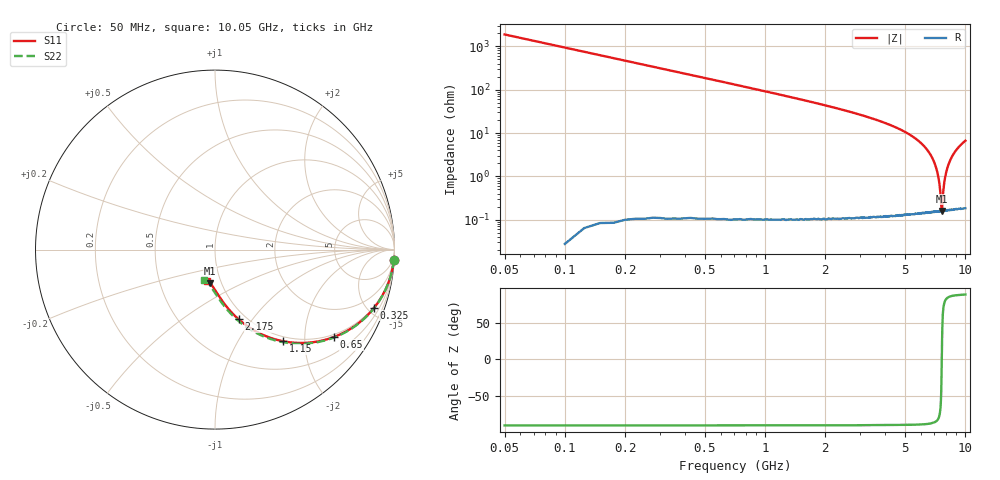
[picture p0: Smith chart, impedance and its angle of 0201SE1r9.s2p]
! AVX Thin Film Operation		Date: August 2001
! Description: Accu-P® Series, Thin Film, SMD, RF Capacitor
! Part Number: 02013J1R9ABW
! 50 MHz  -  10.05 GHz
! Serial Measurements
# mhz S db R 50
!	S11		S21		S12		S22
!	dB	Phase	dB	Phase	dB	Phase	dB	Phase
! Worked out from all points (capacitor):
!   401 points, 50 MHz to 10.05 GHz, reference 50 ohm
!   read as one part in series: C = 1.7 pF near 100 MHz
!   lowest |Z| = 159 mohm at 7.65 GHz (marker M1)
!   series resonance near 7.657 GHz, so ESL is about 250 pH
!   S11 on the Smith chart (normalised r, x): 50 MHz: 1, -36; 325 MHz: 0.92, -5.52; 650 MHz: 0.92, -2.77; 1.15 GHz: 0.92, -1.58; 2.175 GHz: 0.92, -0.86; 10.05 GHz: 0.86, -0.31
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50  -0.01 -3.2  -25.45 86.8  -25.45 86.8  -0.01 -3.2
75  -0.03 -4.8  -21.94 85.2  -21.94 85.2  -0.03 -4.8
125  -0.08 -7.9  -17.55 82.0  -17.55 82.0  -0.08 -8.0
175  -0.15 -11.1  -14.71 78.9  -14.71 78.9  -0.15 -11.1
250  -0.30 -15.6  -11.76 74.3  -11.76 74.3  -0.30 -15.7
325  -0.50 -20.0  -9.68 69.9  -9.68 69.9  -0.50 -20.2
400  -0.73 -24.2  -8.12 65.7  -8.12 65.7  -0.73 -24.4
475  -1.00 -28.1  -6.89 61.7  -6.89 61.7  -1.00 -28.4
650  -1.71 -36.4  -4.89 53.4  -4.89 53.4  -1.70 -36.7
875  -2.71 -45.1  -3.35 44.6  -3.35 44.6  -2.71 -45.6
1150  -3.94 -53.4  -2.25 36.2  -2.25 36.2  -3.94 -54.1
1425  -5.10 -59.8  -1.61 29.7  -1.61 29.7  -5.10 -60.6
1725  -6.25 -65.2  -1.19 24.2  -1.19 24.2  -6.25 -66.2
2175  -7.74 -71.3  -0.81 18.0  -0.81 18.0  -7.74 -72.5
2725  -9.23 -76.6  -0.56 12.4  -0.56 12.4  -9.23 -78.2
3400  -10.66 -81.5  -0.40 7.3  -0.40 7.3  -10.67 -83.4
4175  -11.90 -85.8  -0.30 2.8  -0.30 2.8  -11.91 -88.1
5050  -12.92 -89.7  -0.24 -1.3  -0.24 -1.3  -12.93 -92.4
6725  -14.10 -95.6  -0.18 -7.8  -0.18 -7.8  -14.12 -99.1
7650  -14.46 -98.4  -0.17 -10.9  -0.17 -10.9  -14.48 -102.4
8400  -14.65 -100.6  -0.17 -13.3  -0.17 -13.3  -14.67 -104.9
10050  -14.82 -105.1  -0.16 -18.2  -0.16 -18.2  -14.85 -110.1
